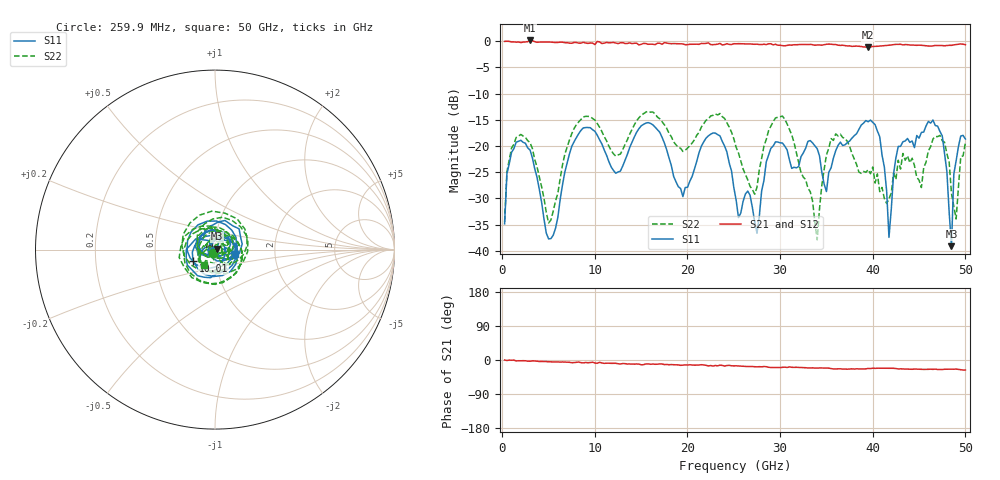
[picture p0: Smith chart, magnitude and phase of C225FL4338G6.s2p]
! 7/2/2020 1:32:39 PM
! D:\C225FL4338G6.S2P
! CHANNEL.1
! TR.MEASUREMENT
! CORRECTED.DATA
# GHZ S RI R 50.0
! FREQ.GHZ  S11RE  S11IM  S21RE  S21IM  S12RE  S12IM  S22RE  S22IM
!; PortSelection: Port_12
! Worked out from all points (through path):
!   200 points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, 259.9 MHz to 50 GHz, reference 50 ohm
!   highest |S21| = 0.15 dB at 3.009 GHz (marker M1); lowest = -1.1 dB at 39.5 GHz (marker M2)
!   group delay of S21, straight-line fit = 1.4 ps
!   lowest |S11| = -39.1 dB at 48.5 GHz (marker M3), VSWR 1.02, Z = 51 + j0.442 ohm
!   |S11| at or under -10 dB: start of sweep to end of sweep
!   |S22| runs from -37.9 to -13.4 dB; largest |S21 - S12| = 0.033
!   S11 on the Smith chart (normalised r, x): 259.9 MHz: 0.98, -0.03; 10.01 GHz: 0.78, -0.10; 50 GHz: 1.25, -0.07
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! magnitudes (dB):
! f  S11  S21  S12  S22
! 259.9 MHz  -34.9  0.0  0.0  -34.5
! 1.01 GHz  -21.2  -0.1  -0.2  -20.4
! 3.009 GHz  -20.8  0.1  0.1  -19.4
! 5.259 GHz  -37.7  -0.2  -0.2  -34.1
! 8.758 GHz  -16.5  -0.2  -0.3  -14.5
! 10.01 GHz  -17.2  -0.6  -0.5  -15.0
! 17.01 GHz  -17.4  -0.4  -0.3  -14.8
! 19.51 GHz  -29.7  -0.5  -0.6  -21.0
! 23.51 GHz  -18.1  -0.4  -0.4  -13.8
! 25.25 GHz  -30.3  -0.5  -0.5  -20.3
! 27.25 GHz  -34.5  -0.6  -0.5  -29.2
! 30.25 GHz  -19.4  -0.8  -0.8  -14.3
! 33.5 GHz  -19.4  -0.7  -0.8  -30.5
! 34 GHz  -20.5  -0.7  -0.7  -37.9
! 36 GHz  -20.9  -0.6  -0.7  -17.7
! 39.5 GHz  -15.4  -1.1  -1.0  -24.5
! 41.75 GHz  -37.4  -0.8  -0.7  -30.1
! 42.75 GHz  -20.1  -0.6  -0.7  -22.7
! 46.5 GHz  -15.0  -0.9  -0.7  -18.6
! 48.5 GHz  -39.1  -0.8  -0.8  -29.1
! 48.75 GHz  -25.4  -0.7  -0.8  -31.5
! 50 GHz  -18.7  -0.7  -0.6  -19.4
